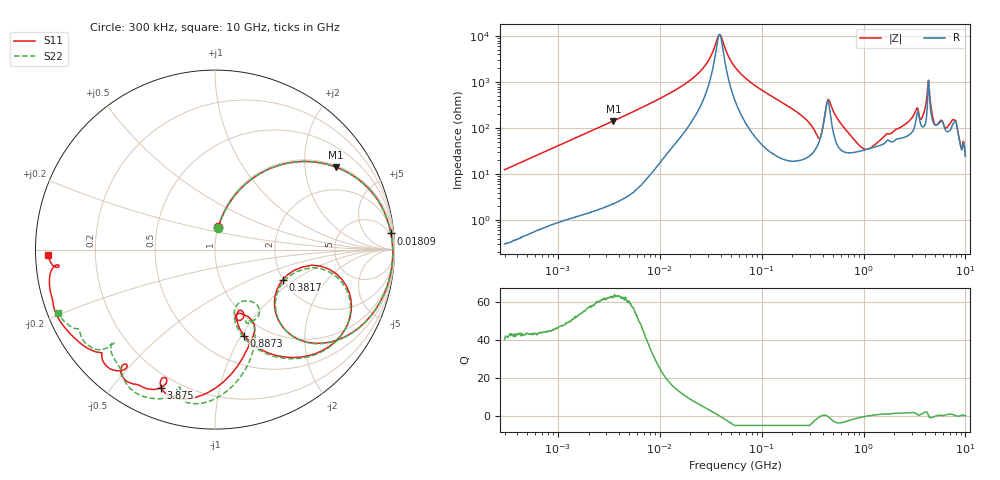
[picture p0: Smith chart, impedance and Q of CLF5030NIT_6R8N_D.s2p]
! S-Parameter Data Generated by TDK Corporation
! Copyright(C) 2019 TDK Corporation.
! All Rights Reserved.
! TDK P/N: CLF5030NIT-6R8N-D (Inductor)
! Property: L=6.8uH at 100kHz
! Size(LxWxT): 5.3x5x2.7mm
! Model Type: s2p (Touchstone File Format Version 1.0)
! Frequency: DC=Yes Start=0.3MHz Stop=10000MHz 802points Log-sweep
! Model Generated on May 10, 2019
! Port Assignments:
!  1 ---@@@--- 2
! Applicable Conditions:
!  Temperature = 25 degC
!  DC Bias Current = 0 A
!  Small Signal Operation
! Terms and conditions regarding TDK Simulation Models
! (1)This simulation model is being provided solely for informational purposes. Please refer to the specifications of the products in terms of detailed characteristics of such products.
! (2)In no event shall TDK Corporation of any of its subsidiaries be liable for any loss or damage arising, directly or indirectly,
!  From any information contained in this simulation model, including, but not limited to loss or damages arising from any inaccuracies, omissions or errors in connection with such information.
! (3)Any and all copyrights on this simulation model are owned by TDK Corporation.
!  Duplication or redistribution of this simulation model without prior written permission from TDK Corporation is prohibited.
! (4)This simulation model is subject to any modification or change without any prior notice.
! (5)Neither TDK Corporation nor any of its subsidiaries shall make any warranty, express or implied,
!  Including but not limited to the correctness, implied warranties of merchantability and fitness for a particular purpose with respect to this simulation models.
! (6)The use of this simulation model shall be deemed to have consented to the terms and conditions hereof.
# Hz S MA R 50
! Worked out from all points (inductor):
!   801 points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, 300 kHz to 10 GHz, reference 50 ohm
!   read as one part in series: L = 6.63 uH near 318.3 kHz
!   highest Q = 62.9 at 3.509 MHz (marker M1), where L = 6.52 uH
!   self-resonance near 38.61 MHz
!   S11 on the Smith chart (normalised r, x): 300 kHz: 1.01, +0.25; 18.09 MHz: 4, +21; 381.7 MHz: 2.00, -0.81; 887.3 MHz: 0.80, -1.03; 3.875 GHz: 0.14, -0.67; 10 GHz: 0.04, -0.02
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300000  0.1245 81.5  0.989 -7.1  0.9889 -7.1  0.1244 81.6
1713600  0.5688 54.2  0.812 -34.7  0.8119 -34.7  0.5689 54.2
3509086  0.8145 34.4  0.5672 -54.7  0.5674 -54.7  0.8146 34.4
9671944  0.9649 12.8  0.2283 -75.0  0.2283 -75.0  0.965 12.8
1.80882e7  0.9844 5.2  0.1044 -79.2  0.1045 -79.2  0.9845 5.2
2.756802e7  0.9892 1.4  0.04458 -76.0  0.04459 -76.0  0.9893 1.4
3.817206e7  0.9907 -1.4  0.009294 -11.4  0.009295 -11.5  0.9908 -1.5
5.477226e7  0.9902 -4.8  0.0466 74.4  0.04662 74.4  0.9903 -4.9
1.720721e8  0.9414 -23.4  0.2842 63.0  0.2842 63.0  0.9415 -23.5
3.126428e8  0.6947 -46.6  0.5745 29.9  0.5745 29.9  0.6956 -46.7
3.816958e8  0.4133 -23.8  0.5896 -9.3  0.5896 -9.3  0.4231 -24.4
4.568044e8  0.8324 -24.3  0.1942 11.5  0.1943 11.5  0.8346 -25.6
5.82867e8  0.7742 -50.4  0.4757 25.8  0.4758 25.8  0.7711 -51.7
8.872678e8  0.5055 -71.3  0.6636 -8.6  0.6638 -8.6  0.4918 -72.8
1.767019e9  0.3834 -72.6  0.5358 -69.3  0.5355 -69.3  0.447 -58.4
2.477118e9  0.6273 -76.1  0.4134 -108.8  0.4127 -108.9  0.6064 -69.7
3.874538e9  0.8268 -111.3  0.1465 -152.3  0.1444 -152.3  0.8374 -105.1
4.34106e9  0.8666 -119.5  0.02242 -116.6  0.02307 -110.0  0.9035 -113.8
5.157474e9  0.8121 -128.3  0.1438 -105.5  0.1454 -105.8  0.8497 -128.3
6.979804e9  0.9001 -142.5  0.08585 -164.0  0.08572 -164.8  0.8483 -138.9
7.875699e9  0.9545 -157.2  0.0332 -155.1  0.03309 -155.1  0.8791 -149.6
1e10  0.929 -178.1  0.0295 -103.9  0.02934 -103.5  0.943 -157.9
